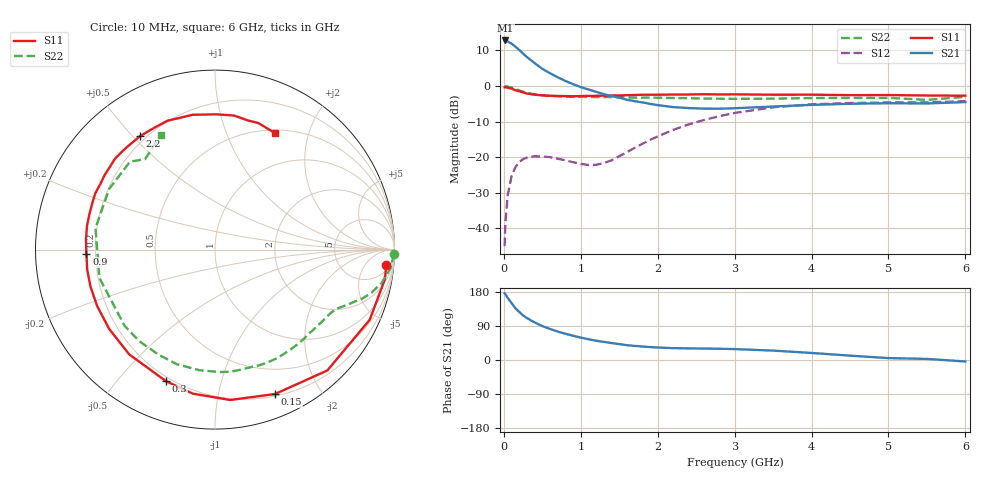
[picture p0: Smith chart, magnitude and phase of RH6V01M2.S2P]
! SIEMENS Small Signal Semiconductors
! BFR106
! Si NPN RF Bipolar Junction Transistor in SOT23
! VCE = 6 V  IC = 1.2 mA
! Common Emitter S-Parameters:  August  1996
# GHz  S  MA  R  50
!  f  S11  S21  S12  S22
! GHz  MAG  ANG  MAG  ANG  MAG  ANG  MAG  ANG
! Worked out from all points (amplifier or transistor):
!   36 points, 10 MHz to 6 GHz, reference 50 ohm
!   highest |S21| = 12.8 dB at 20 MHz (marker M1)
!   |S21| within 3 dB of that: start of sweep to 216.4 MHz
!   unconditionally stable (mu >= 1): 845.8 MHz to 1.826 GHz; 3.333 GHz to end of sweep
!   at 250 MHz: K = 0.27, MSG = 14.8 dB, |S12| = -20.6 dB
!   at 1.4 GHz: K = 1.35, MAG = 5.5 dB, |S12| = -20.9 dB
!   at 6 GHz: K = 1.02, MAG = -1.0 dB, |S12| = -4.3 dB
!   S11 on the Smith chart (normalised r, x): 10 MHz: 9, -19; 150 MHz: 0.22, -1.48; 300 MHz: 0.18, -0.68; 900 MHz: 0.17, -0.02; 2.2 GHz: 0.18, +0.52; 6 GHz: 0.54, +1.50
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0.01  0.9584 -5.0  4.336 176.1  0.0056 90.3  0.9998 -1.4
0.02  0.9609 -9.9  4.361 173.8  0.0117 86.2  0.9931 -2.5
0.05  0.9465 -24.4  4.224 163.8  0.029 75.7  0.9828 -6.1
0.1  0.9193 -47.1  3.934 150.3  0.0537 65.0  0.9469 -11.3
0.15  0.8713 -67.4  3.57 136.7  0.0722 53.6  0.9036 -15.5
0.2  0.8423 -84.2  3.206 126.9  0.0852 45.9  0.8647 -18.4
0.25  0.8121 -98.7  2.857 117.7  0.0937 38.7  0.8279 -20.6
0.3  0.7823 -110.4  2.551 110.7  0.0986 34.3  0.8019 -22.4
0.4  0.7545 -129.3  2.096 99.1  0.1028 27.0  0.7617 -25.3
0.5  0.7369 -143.1  1.741 89.5  0.1023 22.6  0.7385 -28.1
0.7  0.7237 -163.6  1.327 75.1  0.0949 20.2  0.7176 -34.3
0.9  0.7167 -178.1  1.059 64.0  0.0848 24.9  0.7038 -40.9
1.1  0.7253 169.4  0.892 54.8  0.0775 37.1  0.7001 -48.5
1.6  0.7421 145.9  0.64 39.1  0.1173 73.1  0.6904 -69.0
2.2  0.7576 123.5  0.505 31.3  0.2411 75.1  0.6776 -97.3
2.8  0.7595 104.7  0.479 29.7  0.3757 61.6  0.6621 -129.5
3.5  0.7537 89.4  0.514 24.8  0.501 43.0  0.663 -166.2
4  0.7544 81.9  0.542 18.6  0.5525 30.4  0.6765 169.8
4.5  0.7427 75.8  0.562 11.5  0.5755 19.5  0.6796 150.1
5  0.7451 71.1  0.572 5.0  0.5861 10.7  0.6813 134.0
5.5  0.7342 66.0  0.568 2.9  0.5858 6.4  0.6369 127.7
6  0.7304 63.0  0.593 -3.9  0.6129 -1.8  0.7043 115.4
